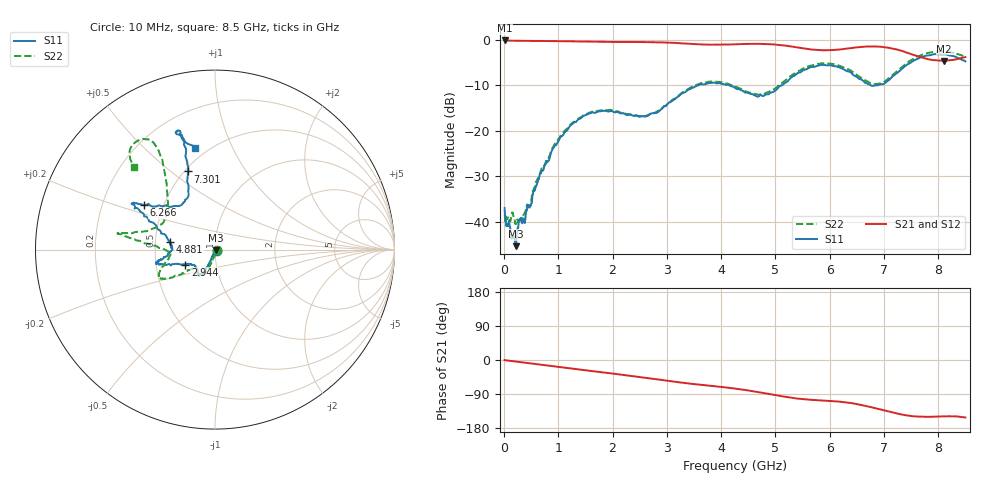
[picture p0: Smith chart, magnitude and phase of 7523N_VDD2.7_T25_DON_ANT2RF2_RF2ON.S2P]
!Agilent Technologies,E5071C,MY46417908,A.11.23
!Date: Wed Dec 09 17:50:04 2020
!Data & Calibration Information:
!Freq	S11:SOLT2(ON)	S21:SOLT2(ON)	S12:SOLT2(ON)	S22:SOLT2(ON)
!PortZ  Port1:50+j0  Port2:50+j0
!Above PortZ is port z conversion or system Z0 setting when saving the data.
!When reading, reference impedance value at option line is always used.
# Hz S dB R 50
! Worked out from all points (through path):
!   1601 points, 10 MHz to 8.5 GHz, reference 50 ohm
!   highest |S21| = -0.17 dB at 10 MHz (marker M1); lowest = -4.6 dB at 8.107 GHz (marker M2)
!   group delay of S21, straight-line fit = 52.1 ps
!   lowest |S11| = -45.3 dB at 216.9 MHz (marker M3), VSWR 1.01, Z = 50.3 - j0.423 ohm
!   |S11| at or under -10 dB: start of sweep to 3.584 GHz; 4.149 GHz to 5.12 GHz (970.6 MHz wide, 20.9 % of centre); 6.753 GHz to 6.876 GHz (123.7 MHz wide, 1.82 % of centre)
!   |S22| runs from -40.5 to -2.6 dB; largest |S21 - S12| = 0.0039
!   S11 on the Smith chart (normalised r, x): 10 MHz: 1.03, -0.01; 2.944 GHz: 0.71, -0.12; 4.881 GHz: 0.60, +0.06; 6.266 GHz: 0.39, +0.25; 7.301 GHz: 0.52, +0.58; 8.5 GHz: 0.43, +0.73
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1e7  -36.95 -23.2  -0.17 -0.3  -0.17 -0.3  -38.41 -2.1
1.744938e8  -43.29 -54.0  -0.23 -3.4  -0.23 -3.4  -38.76 -32.5
2.169438e8  -45.33 -50.9  -0.24 -4.2  -0.24 -4.2  -40.29 -46.5
2.85925e8  -39.61 -71.4  -0.24 -5.4  -0.24 -5.4  -39.58 -70.6
4.716438e8  -36.60 -96.8  -0.26 -8.8  -0.26 -8.8  -36.85 -83.6
6.520562e8  -29.93 -110.5  -0.29 -12.0  -0.29 -12.0  -29.90 -93.9
9.0145e8  -23.87 -110.2  -0.32 -16.5  -0.32 -16.5  -23.69 -105.3
1.426769e9  -17.10 -116.3  -0.41 -25.9  -0.40 -26.0  -16.92 -114.4
1.83535e9  -15.63 -123.5  -0.48 -32.9  -0.48 -32.9  -15.41 -120.9
2.843538e9  -15.81 -150.5  -0.58 -51.4  -0.58 -51.4  -15.65 -140.2
2.944356e9  -14.67 -152.8  -0.61 -53.4  -0.62 -53.4  -14.66 -142.0
3.607638e9  -9.86 -165.5  -1.03 -65.2  -1.03 -65.2  -9.61 -150.3
4.255e9  -10.58 -169.7  -1.01 -75.5  -1.00 -75.5  -10.28 -162.2
4.881138e9  -11.91 170.2  -0.98 -89.7  -0.98 -89.6  -11.45 -178.5
5.671769e9  -5.96 152.8  -2.17 -105.2  -2.16 -105.0  -5.62 170.8
6.266069e9  -6.58 148.1  -2.03 -111.2  -2.03 -111.2  -6.15 169.1
6.775469e9  -10.11 127.9  -1.49 -124.9  -1.48 -124.9  -9.65 154.6
7.088538e9  -8.87 114.4  -1.78 -136.1  -1.78 -136.3  -8.50 134.2
7.300788e9  -6.73 109.0  -2.36 -143.1  -2.35 -143.2  -6.31 124.7
7.719981e9  -3.73 106.2  -3.99 -149.7  -4.00 -149.7  -3.22 120.0
8.107338e9  -3.21 107.9  -4.65 -148.6  -4.67 -148.5  -2.57 127.2
8.5e9  -4.76 101.1  -3.82 -151.7  -3.82 -151.5  -3.80 134.3
